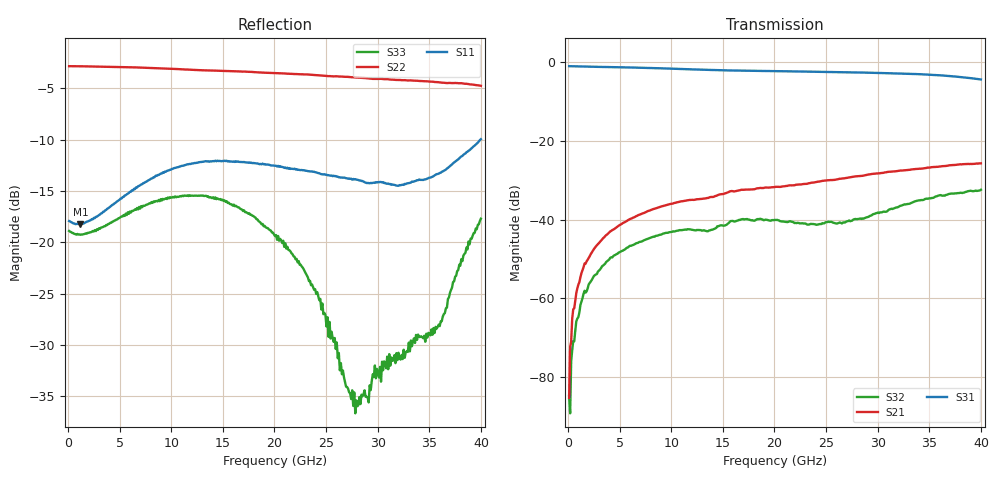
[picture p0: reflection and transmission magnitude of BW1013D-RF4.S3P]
!  3-Port S-parameters saved by WinCal
! VAR MeasName=S-Parameters (CALIBRATED_DATA) read from VNA (N5245A)
! VAR MeasDate=12/26/2016 18:40:45
! VAR NAME=158306_25-RF4
! VAR FILENAME=158306_25-RF4.S3P
! VAR DATE=12/26/2016 18:40:45
! VAR PHYS_PORTS=1,2,3
# Hz S RI R 50
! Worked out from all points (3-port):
!   401 points, 100 MHz to 40 GHz, reference 50 ohm
!   strongest paths, dB at 100 MHz, 10.07 GHz, 20.05 GHz, 30.02 GHz, 40 GHz:
!     S31: -1.1, -1.8, -2.4, -2.8, -4.5
!     S21: -85.2, -36.0, -31.8, -28.3, -25.8
!     S32: -84.7, -43.1, -40.1, -38.2, -32.5
!   lowest |S11| = -18.2 dB at 1.197 GHz (marker M1), VSWR 1.28, Z = 62.6 - j5.71 ohm
!   |S11| at or under -10 dB: start of sweep to 39.96 GHz
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1e8  0.1268 -0.00575  2.86e-05 6.36e-05  0.8764 -0.0115
     -1.96e-06 5.5e-05  -0.72 0.00268  -3.83e-05 3.05e-05
     0.8768 -0.0114  1.11e-05 -5.73e-05  0.1134 -0.00468
4.99e8  0.1217 -0.022  -0.000155 0.000679  0.871 -0.0503
        -0.000119 0.000721  -0.7198 0.0129  -0.000132 0.000264
        0.8714 -0.0503  -8.87e-05 0.000275  0.1094 -0.0182
1.19725e9  0.114 -0.045  -0.000195 0.00188  0.8593 -0.1125
           -0.000229 0.00186  -0.7185 0.0303  -0.000206 0.00077
           0.8599 -0.1124  -0.000246 0.000793  0.1022 -0.0372
2.893e9  0.0948 -0.0956  0.000655 0.0049  0.8203 -0.2543
         0.000696 0.00484  -0.7133 0.0712  0.0003 0.00218
         0.8207 -0.2542  0.00032 0.00217  0.0839 -0.0784
5.98525e9  0.0329 -0.173  0.00439 0.00912  0.6917 -0.483
           0.00442 0.00911  -0.6971 0.1425  0.00268 0.00373
           0.6924 -0.4832  0.00276 0.00374  0.0256 -0.1389
1.276825e10  -0.149 -0.1952  0.0156 0.00931  0.236 -0.756
             0.0156 0.00933  -0.6273 0.2845  0.00733 0.000508
             0.2363 -0.7566  0.00734 0.0005  -0.1214 -0.1168
2.005e10  -0.2211 -0.0823  0.0258 0.00063  -0.2832 -0.7025
          0.0258 0.000689  -0.5198 0.4168  0.00774 -0.00607
          -0.2834 -0.7036  0.00776 -0.00614  -0.1072 0.00279
2.803e10  -0.1978 0.0383  0.0301 -0.0183  -0.6776 -0.2687
          0.0302 -0.0183  -0.349 0.5289  0.00486 -0.00894
          -0.6785 -0.2685  0.0048 -0.00892  -0.0118 -0.0106
3.601e10  -0.00413 0.2174  0.0101 -0.046  -0.5727 0.3503
          0.00999 -0.046  -0.131 0.5862  -0.00661 -0.0192
          -0.5736 0.3508  -0.00673 -0.0192  0.0289 -0.0263
4e10  0.2535 0.1914  -0.0145 -0.0496  -0.2893 0.5193
      -0.0146 -0.0494  -0.00392 0.5779  -0.019 -0.0143
      -0.2896 0.5202  -0.019 -0.0144  0.1129 -0.0651
